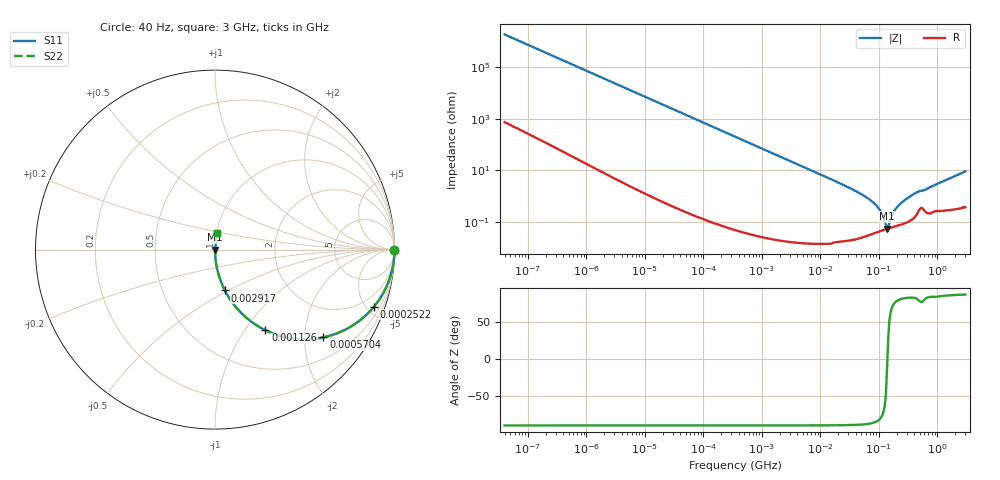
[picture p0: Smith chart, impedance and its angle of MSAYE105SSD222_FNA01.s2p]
! MSAYE105SSD222_FNA01  S-PARAMETER MODEL  ( General Type )
! Model Generated by TAIYO YUDEN Corporation (http://www.ty-top.com)
! Version 2.0
! TAIYO YUDEN Control No. 040624
! Copyright(c) 2004 TAIYO YUDEN CO.,LTD. All Rights Reserved.
! Product Description (link to TY-COMPAS)
! https://ds.yuden.co.jp/TYCOMPAS/or/detail?pn=MSAYE105SSD222KFNA01&u=M
! Products Name : Multilayer Ceramic Capacitors
! Characteristics :
!  Capacitance : 2200 pF , Rated Voltage : 16V
!  Case Size : 1.0 x 0.5 / 0.039 x 0.02 [mm/inch] , Thickness : 0.5 / 0.02 [mm/inch]
!  (Conditions: Temperature = 25 degC , DC Bias Current/Voltage = 0A / 0V)
! External Node Assignments :
!  1  o---| |---o  2
! GND o---------o GND
! Frequency Range : 40Hz  -  3GHz  [ 401 STEP ]
# MHz S RI R 50
! Freq[MHz].  S11 Real  S11 Imag  S21 Real  S21 Imag  S12 Real  S12 Imag  S22 Real  S22 Imag
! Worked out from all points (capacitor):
!   401 points, 40 Hz to 3 GHz, reference 50 ohm
!   read as one part in series: C = 2.26 nF near 44 Hz
!   lowest |Z| = 57.4 mohm at 137.5 MHz (marker M1)
!   series resonance near 139.4 MHz, so ESL is about 580 pH
!   S11 on the Smith chart (normalised r, x): 40 Hz: open; 252.2 kHz: 1.00, -5.58; 570.4 kHz: 1.00, -2.47; 1.126 MHz: 1.00, -1.25; 2.917 MHz: 1.00, -0.48; 3 GHz: 1.01, +0.18
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4e-05  1 -5.68e-05  2.7e-08 5.68e-05  2.7e-08 5.68e-05  1 -5.68e-05
7.9e-05  1 -0.000112  5.6e-08 0.000112  5.6e-08 0.000112  1 -0.000112
0.000834  1 -0.00119  1.71e-06 0.00119  1.71e-06 0.00119  1 -0.00119
0.017386  0.9994 -0.0247  0.000614 0.0247  0.000614 0.0247  0.9994 -0.0247
0.081206  0.9868 -0.1139  0.0132 0.1139  0.0132 0.1139  0.9868 -0.1139
0.252219  0.8861 -0.3176  0.1139 0.3176  0.1139 0.3176  0.8861 -0.3176
0.362475  0.7903 -0.407  0.2097 0.407  0.2097 0.407  0.7903 -0.407
0.570368  0.6035 -0.489  0.3965 0.489  0.3965 0.489  0.6035 -0.489
1.125822  0.281 -0.4493  0.719 0.4493  0.719 0.4493  0.281 -0.4493
2.916825  0.0551 -0.2278  0.9449 0.2278  0.9449 0.2278  0.0551 -0.2278
7.222098  0.0095 -0.0962  0.9905 0.0962  0.9905 0.0962  0.0095 -0.0962
32.2371  0.000622 -0.0206  0.9994 0.0206  0.9994 0.0206  0.000622 -0.0206
66.58224  0.000379 -0.00805  0.9996 0.00805  0.9996 0.00805  0.000379 -0.00805
100.1261  0.000451 -0.00333  0.9995 0.00333  0.9995 0.00333  0.000451 -0.00333
131.4235  0.000542 -0.000583  0.9995 0.000583  0.9995 0.000583  0.000542 -0.000583
137.5184  0.00056 -0.000125  0.9994 0.000125  0.9994 0.000125  0.00056 -0.000125
150.5692  0.000597 0.000756  0.9994 -0.000756  0.9994 -0.000756  0.000597 0.000756
172.504  0.000657 0.00209  0.9993 -0.00209  0.9993 -0.00209  0.000657 0.00209
197.6342  0.000725 0.00345  0.9993 -0.00345  0.9993 -0.00345  0.000725 0.00345
325.4065  0.00117 0.00925  0.9988 -0.00925  0.9988 -0.00925  0.00117 0.00925
467.657  0.00271 0.015  0.9973 -0.015  0.9973 -0.015  0.00271 0.015
3000  0.012 0.0902  0.988 -0.0902  0.988 -0.0902  0.012 0.0902
